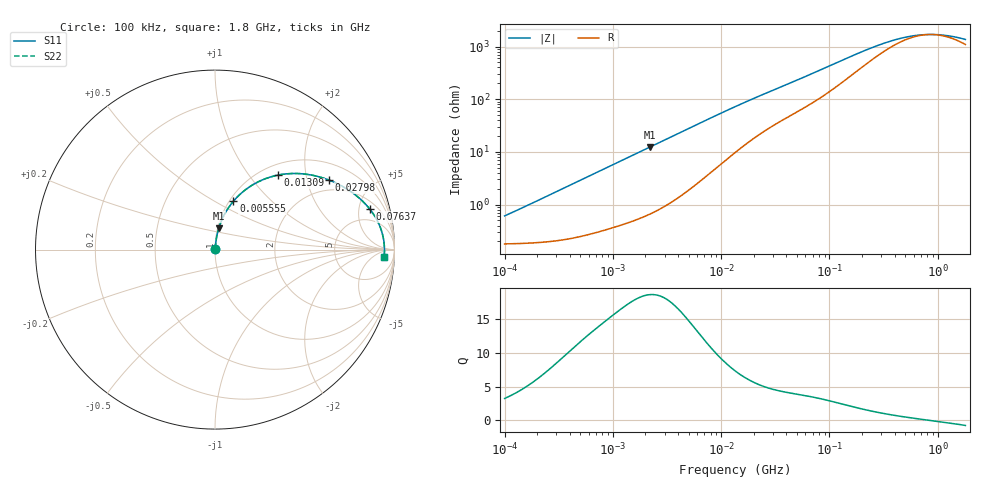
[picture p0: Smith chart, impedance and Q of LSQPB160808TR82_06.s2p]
! LSQPB160808TR82_06  S-PARAMETER MODEL  ( General Type )
! Model Generated by TAIYO YUDEN Corporation (http://www.ty-top.com)
! Version 1.0
! TAIYO YUDEN Control No. 110726NG25SE-FKC
! Copyright(c) 2011 TAIYO YUDEN CO.,LTD. All Rights Reserved.
! Product Description (link to TY-COMPAS)
! https://ds.yuden.co.jp/TYCOMPAS/or/detail?pn=LSQPB160808TR82M06&u=M
! Products Name : Inductors
! Characteristics :
!  Inductance : 0.82 uH , SRF(min) : 560 MHz , DC Resistance(max) : 0.2288 Ohm
!  Rated Current : Saturation :950 mA , Temp Rise : 730 mA (40 degC)
!  Case Size : 1.6 x 0.8 / 0.063 x 0.031 [mm/inch] , Thickness : 0.8 / 0.031 [mm/inch]
!  (Conditions: Temperature = 25 degC , DC Bias Current/Voltage = 0A / 0V)
! External Node Assignments :
!  1  o---GGG---o  2
! GND o---------o GND
! Frequency Range : 0.1MHz  -  1800MHz  [ 402 STEP ]
# MHz S RI R 50
! Freq[MHz].  S11 Real  S11 Imag  S21 Real  S21 Imag  S12 Real  S12 Imag  S22 Real  S22 Imag
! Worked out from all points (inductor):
!   401 points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, 100 kHz to 1.8 GHz, reference 50 ohm
!   read as one part in series: L = 929 nH near 105 kHz
!   highest Q = 18.6 at 2.19 MHz (marker M1), where L = 893 nH
!   self-resonance near 855.4 MHz
!   S11 on the Smith chart (normalised r, x): 100 kHz: 1.00, +0.01; 5.555 MHz: 1.04, +0.62; 13.09 MHz: 1.19, +1.40; 27.98 MHz: 1.57, +2.72; 76.37 MHz: 2.92, +6.43; 1.8 GHz: 23, -16
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0.1  0.00183 0.00582  0.9982 -0.00582  0.9982 -0.00582  0.00183 0.00582
0.516129  0.00339 0.0296  0.9966 -0.0296  0.9966 -0.0296  0.00339 0.0296
1.158292  0.00824 0.0649  0.9918 -0.0649  0.9918 -0.0649  0.00824 0.0649
2.189832  0.0211 0.1195  0.9789 -0.1195  0.9789 -0.1195  0.0211 0.1195
2.66389  0.0292 0.1436  0.9708 -0.1436  0.9708 -0.1436  0.0292 0.1436
3.942096  0.0573 0.2043  0.9427 -0.2043  0.9427 -0.2043  0.0573 0.2043
5.554714  0.1029 0.2699  0.8971 -0.2699  0.8971 -0.2699  0.1029 0.2699
8.423854  0.1984 0.3537  0.8016 -0.3537  0.8016 -0.3537  0.1984 0.3537
13.09176  0.3502 0.4149  0.6498 -0.4149  0.6498 -0.4149  0.3502 0.4149
13.41641  0.3596 0.4167  0.6404 -0.4167  0.6404 -0.4167  0.3596 0.4167
18.90474  0.4938 0.4217  0.5062 -0.4217  0.5062 -0.4217  0.4938 0.4217
27.97575  0.6331 0.3881  0.3669 -0.3881  0.3669 -0.3881  0.6331 0.3881
43.47794  0.7567 0.3233  0.2433 -0.3233  0.2433 -0.3233  0.7567 0.3233
69.24595  0.8475 0.2435  0.1525 -0.2435  0.1525 -0.2435  0.8475 0.2435
76.37428  0.8616 0.2268  0.1384 -0.2268  0.1384 -0.2268  0.8616 0.2268
144.3909  0.9181 0.1311  0.0819 -0.1311  0.0819 -0.1311  0.9181 0.1311
241.5136  0.9353 0.0767  0.0647 -0.0767  0.0647 -0.0767  0.9353 0.0767
357.3983  0.9408 0.047  0.0592 -0.047  0.0592 -0.047  0.9408 0.047
542.0029  0.9433 0.0226  0.0567 -0.0226  0.0567 -0.0226  0.9433 0.0226
802.0705  0.9442 0.00308  0.0558 -0.00308  0.0558 -0.00308  0.9442 0.00308
1186.925  0.9441 -0.016  0.0559 0.016  0.0559 0.016  0.9441 -0.016
1800  0.9428 -0.039  0.0572 0.039  0.0572 0.039  0.9428 -0.039
